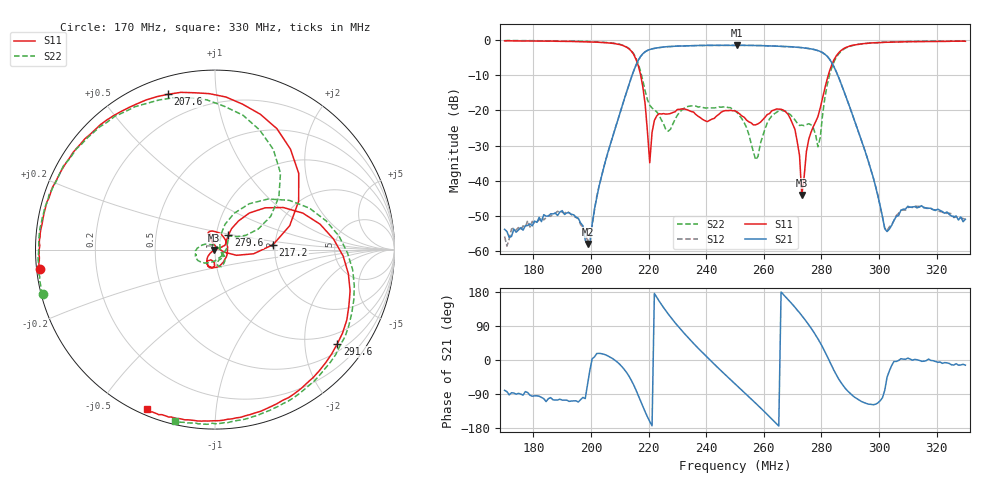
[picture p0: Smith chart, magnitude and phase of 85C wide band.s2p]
!Agilent Technologies,E8362C,SG49020144,A.09.33.09
!Agilent E8362C: A.09.33.09
!Date: Friday, October 10, 2025 10:36:41
!Correction: S11(Full 2 Port(1,2))
!S21(Full 2 Port(1,2))
!S12(Full 2 Port(1,2))
!S22(Full 2 Port(1,2))
!S2P File: Measurements: S11, S21, S12, S22:
# Hz S  dB  R 50
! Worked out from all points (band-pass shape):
!   201 points, 170 MHz to 330 MHz, reference 50 ohm
!   highest |S21| = -1.41 dB at 250.8 MHz (marker M1); lowest = -58.0 dB at 198.8 MHz (marker M2)
!   |S21| within 3 dB of the highest: 217.4 MHz to 281.8 MHz (64.44 MHz wide, 25.8 % of centre)
!   lowest |S11| = -44.1 dB at 273.2 MHz (marker M3), VSWR 1.01, Z = 49.4 - j0.267 ohm
!   |S11| at or under -10 dB: 217.3 MHz to 282.4 MHz (65.12 MHz wide, 26.1 % of centre)
!   |S22| runs from -34.1 to 0.0 dB; largest |S21 - S12| = 0.0059
!   S11 on the Smith chart (normalised r, x): 170 MHz: 0.01, -0.05; 207.6 MHz: 0.08, +0.74; 217.2 MHz: 1.95, +0.12; 279.6 MHz: 1.14, +0.18; 291.6 MHz: 0.69, -2.78; 330 MHz: 0.02, -0.66
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1.7e8  -0.16 -173.7  -53.88 -80.2  -55.92 -84.5  -0.09 -165.5
1.972e8  -0.40 143.7  -52.88 -98.8  -53.20 -99.6  -0.33 155.1
1.988e8  -0.42 139.6  -58.02 -63.8  -57.03 -64.6  -0.31 150.8
2.076e8  -0.87 106.9  -27.23 3.4  -27.29 3.1  -0.79 119.3
2.132e8  -2.42 62.9  -12.55 -42.8  -12.52 -43.0  -2.33 78.2
2.172e8  -9.76 4.9  -4.62 -108.1  -4.65 -108.1  -8.84 30.8
2.204e8  -34.91 78.5  -2.63 -162.3  -2.63 -162.5  -18.51 39.2
2.236e8  -20.92 107.4  -2.08 156.1  -2.09 156.1  -21.24 33.4
2.3e8  -19.72 111.2  -1.66 91.1  -1.66 91.4  -21.35 -119.6
2.38e8  -22.07 40.7  -1.45 25.0  -1.47 24.8  -18.92 -163.6
2.5e8  -20.10 -111.6  -1.44 -62.7  -1.43 -62.8  -20.10 175.0
2.508e8  -20.45 -116.2  -1.41 -68.5  -1.43 -68.5  -20.65 172.6
2.572e8  -24.09 -106.7  -1.47 -114.3  -1.50 -114.5  -34.09 62.8
2.684e8  -21.08 -120.3  -1.81 160.0  -1.82 159.9  -20.75 -80.4
2.716e8  -28.85 -141.9  -1.98 131.8  -1.99 132.0  -23.58 -74.6
2.732e8  -44.12 -154.3  -2.08 117.2  -2.13 117.2  -24.17 -60.6
2.772e8  -24.59 22.8  -2.58 75.3  -2.59 75.2  -24.98 -39.1
2.796e8  -19.28 47.2  -3.17 45.3  -3.22 45.3  -27.70 49.8
2.836e8  -7.00 31.6  -6.37 -15.5  -6.42 -15.3  -7.76 43.6
2.916e8  -1.31 -37.6  -23.04 -98.5  -23.08 -98.6  -1.33 -29.7
3.036e8  -0.54 -77.9  -53.83 -28.9  -53.18 -27.9  -0.51 -69.7
3.3e8  -0.28 -113.1  -51.00 -13.6  -51.02 -14.6  -0.17 -103.3
